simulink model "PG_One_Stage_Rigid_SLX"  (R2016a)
settings: Solver=ode45  StartTime=0.0  StopTime=10.0  MaxStep=0.001  RelTol=1e-3
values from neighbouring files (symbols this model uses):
  A = eval(A)    [PG_One_Stage_Elastic.m]    (also in PG_One_Stage_Rigid.m = eval(A1))
  B = eval(B)    [PG_One_Stage_Elastic.m]    (also in PG_One_Stage_Rigid.m = eval(B1))
  BQ = BJ*Q    [PG_One_Stage_Rigid.m]
  C = eval(C)    [PG_One_Stage_Elastic.m]    (also in PG_One_Stage_Rigid.m = eval(C1))
  CF = eval(CF)    [PG_One_Stage_Elastic.m]    (also in PG_One_Stage_Rigid.m = inv(R*R.')*R)
  JQ = J*Q    [PG_One_Stage_Rigid.m]
  L = eval(L)    [PG_One_Stage_Elastic.m]    (also in PG_One_Stage_Rigid.m = eval(L1))
  Tau = [100    0    0    0    0    0]*Nm    [PG_One_Stage_Elastic.m]    (also in PG_One_Stage_Rigid.m)
  Ts = Tfin/Nr_Ts_Points    [PG_One_Stage_Elastic.m]    (also in PG_One_Stage_Rigid.m)
  X_0 = [W_0 F_0]    [PG_One_Stage_Elastic.m]    (also in PG_One_Stage_Rigid.m = [0  0]*rpm)

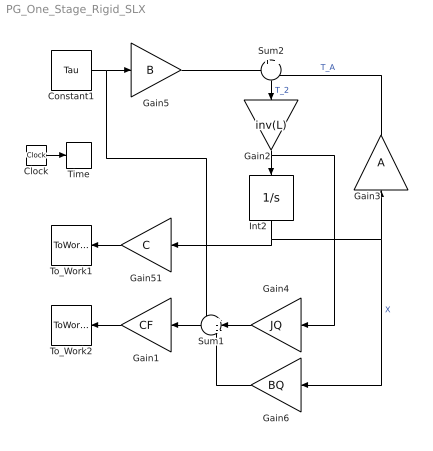
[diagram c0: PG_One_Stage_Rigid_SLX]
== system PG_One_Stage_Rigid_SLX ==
  Clock : Clock
  Constant1 : Constant  Value=Tau  VectorParams1D=off
  Gain1 : Gain  Gain=CF  Multiplication=Matrix(K*u) (u vector)
  Gain2 : Gain  Gain=inv(L)  Multiplication=Matrix(K*u) (u vector)
  Gain3 : Gain  Gain=A  Multiplication=Matrix(K*u) (u vector)
  Gain4 : Gain  Gain=JQ  Multiplication=Matrix(K*u) (u vector)
  Gain5 : Gain  Gain=B  Multiplication=Matrix(K*u) (u vector)
  Gain51 : Gain  Gain=C  Multiplication=Matrix(K*u) (u vector)
  Gain6 : Gain  Gain=BQ  Multiplication=Matrix(K*u) (u vector)
  Int2 : Integrator  InitialCondition=X_0
  Sum1 : Sum  Inputs=+--
  Sum2 : Sum  Inputs=+|+
  Time : ToWorkspace  VariableName=t  SampleTime=Ts
  To_Work1 : ToWorkspace  VariableName=W  SampleTime=Ts
  To_Work2 : ToWorkspace  VariableName=F  SampleTime=Ts
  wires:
  Int2/1 -> Gain51/1, Gain3/1, Gain6/1  "X"
  Sum2/1 -> Gain2/1  "T_2"
  Gain3/1 -> Sum2/2  "T_A"
  Clock/1 -> Time/1
  Constant1/1 -> Sum1/1, Gain5/1
  Gain51/1 -> To_Work1/1
  Gain5/1 -> Sum2/1
  Gain2/1 -> Gain4/1, Int2/1
  Gain1/1 -> To_Work2/1
  Sum1/1 -> Gain1/1
  Gain4/1 -> Sum1/2
  Gain6/1 -> Sum1/3
